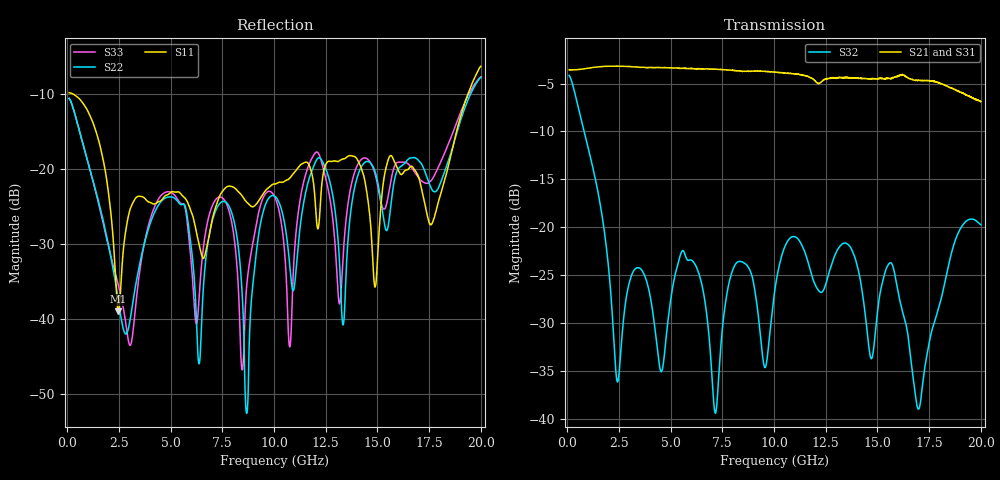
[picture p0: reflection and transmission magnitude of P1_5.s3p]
!The following data was pulled from an Agilent PNA
!This sNp file was generated from the data in the RF Test software
!NOTE:  Smoothing/Math/Corrections applied on any given trace ARE included in the data saved here
# MHz S dB R 50
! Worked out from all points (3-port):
!   6401 points, 100 MHz to 20 GHz, reference 50 ohm
!   strongest paths, dB at 100 MHz, 5.075 GHz, 10.05 GHz, 15.03 GHz, 20 GHz:
!     S21: -3.6, -3.4, -3.8, -4.5, -6.9
!     S31: -3.6, -3.4, -3.8, -4.5, -6.7
!     S32: -4.1, -26.6, -26.5, -28.5, -19.7
!   lowest |S11| = -39.0 dB at 2.485 GHz (marker M1), VSWR 1.02, Z = 49.9 + j1.12 ohm
!   |S11| at or under -10 dB: 239 MHz to 19.38 GHz (19.14 GHz wide, 195 % of centre)
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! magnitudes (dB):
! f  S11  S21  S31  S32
! 100 MHz  -9.9  -3.6  -3.6  -4.1
! 2.485 GHz  -39.0  -3.2  -3.2  -35.8
! 5.184 GHz  -23.1  -3.4  -3.4  -25.4
! 6.384 GHz  -30.1  -3.5  -3.5  -24.9
! 7.684 GHz  -22.5  -3.6  -3.6  -27.5
! 8.679 GHz  -24.5  -3.7  -3.8  -23.9
! 10.05 GHz  -22.0  -3.8  -3.8  -26.5
! 13.34 GHz  -18.7  -4.4  -4.4  -21.7
! 14.89 GHz  -35.7  -4.5  -4.5  -31.2
! 20 GHz  -6.4  -6.9  -6.7  -19.7
